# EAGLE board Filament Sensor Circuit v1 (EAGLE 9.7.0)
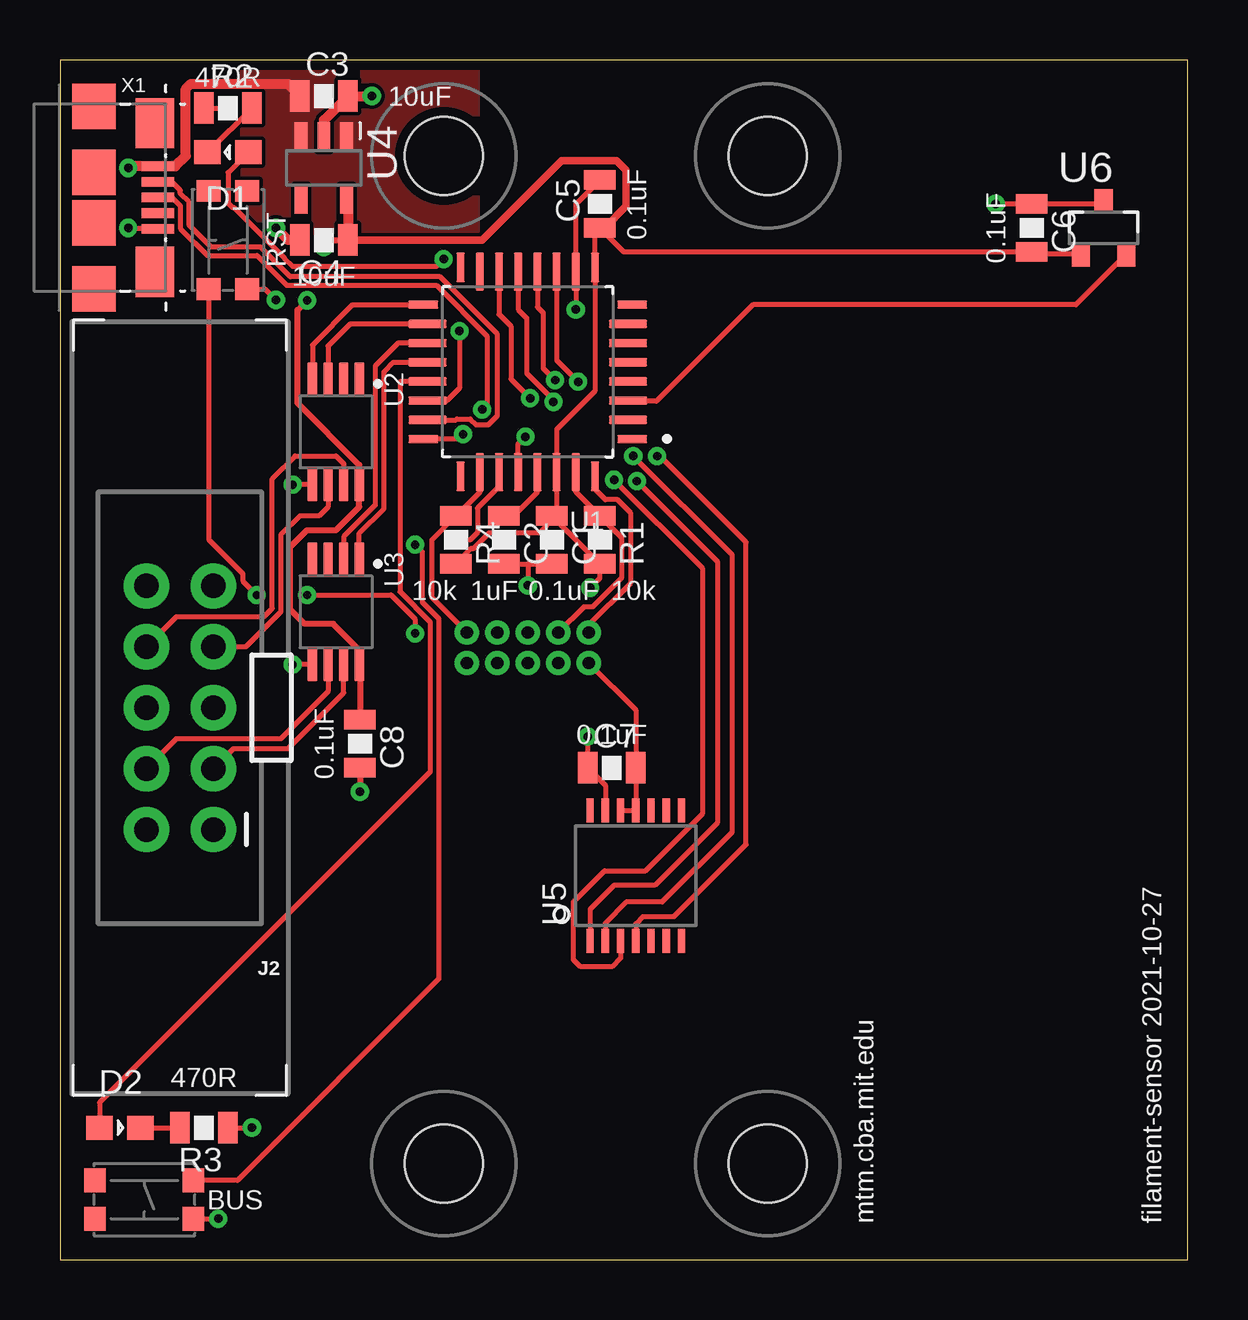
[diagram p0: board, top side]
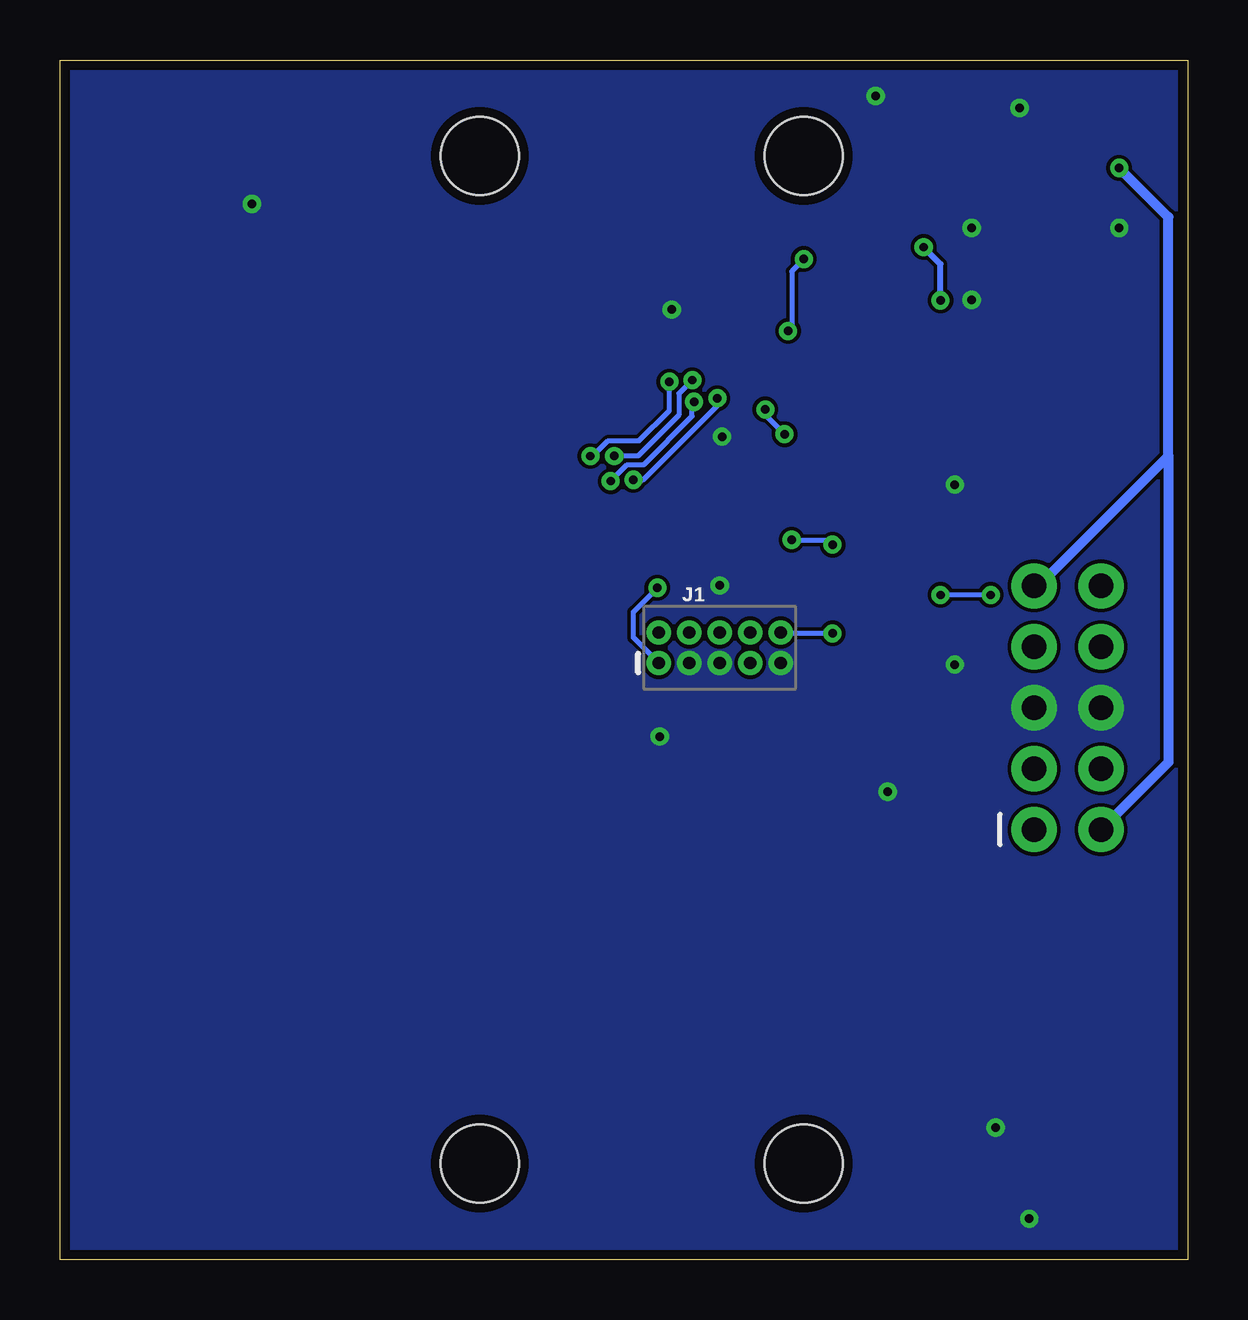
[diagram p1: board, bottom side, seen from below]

Size 47 x 50 mm. Coordinates in mm from the lower left corner, seen from the top.
Outline: 0,0 47,0 47,50 0,50 0,0
Copper layers (1*16): Top 0.035mm / dielectric 1.5mm / Bottom 0.035mm
Design rules "default *": minimum track width 6mil, minimum drill 0.35mm, track to track 6mil, track to pad 6mil, pad to pad 6mil, via to via 6mil, smd to smd 6mil, copper to edge 16mil, drill to drill 6mil, minimum pad ring 10mil, minimum via ring 8mil, stop-mask expansion 4mil, vias tented up to drill 40mil, thermal gap 10mil
Holes 3.25 mm at 16,46 29.5,46 16,4 29.5,4

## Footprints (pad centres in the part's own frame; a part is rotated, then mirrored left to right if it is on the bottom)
0805 = smd 0.8 x 1.3: 1 -1,0; 2 1,0
LED0805 = smd 1.1 x 1: 1 -0.85,0; 2 0.85,0
2X5-PTH-1.27MM = drill 0.508 pad 1: 1 -2.54,-0.635; 2 -2.54,0.635; 3 -1.27,-0.635; 4 -1.27,0.635; 5 0,-0.635; 6 0,0.635; 7 1.27,-0.635; 8 1.27,0.635; 9 2.54,-0.635; 10 2.54,0.635
2X5-SHROUDED_LOCK_LATCH = drill 1.016 pad 1.88: 1 -1.397,5.08; 2 1.397,5.08; 3 -1.397,2.54; 4 1.397,2.54; 5 -1.397,0; 6 1.397,0; 7 -1.397,-2.54; 8 1.397,-2.54; 9 -1.397,-5.08; 10 1.397,-5.08
TACT-SWITCH-KMR6 = smd 0.9 x 1: P$1 -2.05,0.8; P$2 2.05,0.8; P$3 -2.05,-0.8; P$4 2.05,-0.8
TQFP-32-FAB = smd 1.25 x 0.35: 1 -4.355,2.8; 8 -4.355,-2.8; 17 4.355,-2.8; 24 4.355,2.8 | smd 1.6 x 0.35: 2 -4.18,2; 3 -4.18,1.2; 4 -4.18,0.4; 5 -4.18,-0.4; 6 -4.18,-1.2; 7 -4.18,-2; 18 4.18,-2; 19 4.18,-1.2; 20 4.18,-0.4; 21 4.18,0.4; 22 4.18,1.2; 23 4.18,2 | smd 0.35 x 1.25: 9 -2.8,-4.355; 16 2.8,-4.355; 25 2.8,4.355; 32 -2.8,4.355 | smd 0.35 x 1.6: 10 -2,-4.18; 11 -1.2,-4.18; 12 -0.4,-4.18; 13 0.4,-4.18; 14 1.2,-4.18; 15 2,-4.18; 26 2,4.18; 27 1.2,4.18; 28 0.4,4.18; 29 -0.4,4.18; 30 -1.2,4.18; 31 -2,4.18
8-MSOP = smd 1.4 x 0.4: 1 -2.2,0.975; 2 -2.2,0.325; 3 -2.2,-0.325; 4 -2.2,-0.975; 5 2.2,-0.975; 6 2.2,-0.325; 7 2.2,0.325; 8 2.2,0.975
SOT23-5 = smd 0.533 x 1.194: 1 -0.95,-1.306; 2 0,-1.306; 3 0.95,-1.306; 4 0.95,1.306; 5 -0.95,1.306
TSSOP14 = smd 0.305 x 0.991: 1 -1.905,-2.718; 2 -1.27,-2.718; 3 -0.635,-2.718; 4 0,-2.718; 5 0.635,-2.718; 6 1.27,-2.718; 7 1.905,-2.718; 8 1.905,2.718; 9 1.27,2.718; 10 0.635,2.718; 11 0,2.718; 12 -0.635,2.718; 13 -1.27,2.718; 14 -1.905,2.718
SOT23 = smd 0.762 x 1.016: 1 -0.95,-1.1; 2 0.95,-1.1; 3 0,1.1
USB_MICRO_609-4613-1-ND = smd 0.4 x 1.35: D+ 0,2.675; D- -0.65,2.675; GND 1.3,2.675; ID 0.65,2.675; VBUS -1.3,2.675 | smd 1.9 x 1.8: HD0 -3.8,0; HD1 -1.05,0; HD2 1.05,0; HD3 3.8,0 | smd 2.1 x 1.6: HD4 -3.1,2.55; HD5 3.1,2.55

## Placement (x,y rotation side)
C1  0.1uF  [0805]  20.5,30 270 top
C2  1uF  [0805]  18.5,30 270 top
C3  10uF  [0805]  11,48.5 0 top
C4  10uF  [0805]  11,42.5 180 top
C5  0.1uF  [0805]  22.5,44 90 top
C6  0.1uF  [0805]  40.5,43 270 top
C7  0.1uF  [0805]  23,20.5 0 top
C8  0.1uF  [0805]  12.5,21.5 270 top
D1  LED0805  [LED0805]  7,46.15 180 top
D2  LED0805  [LED0805]  2.5,5.5 0 top
J1  CORTEX_DEBUG_PTH  [2X5-PTH-1.27MM]  19.5,25.5 0 bottom
J2  [2X5-SHROUDED_LOCK_LATCH]  5,23 180 top
R1  10k  [0805]  22.5,30 270 top
R2  470R  [0805]  7,48 0 top
R3  470R  [0805]  6,5.5 180 top
R4  10k  [0805]  16.5,30 270 top
S1  2-8X4-5_SWITCH  [TACT-SWITCH-KMR6]  7,42.5 270 top
S2  2-8X4-5_SWITCH  [TACT-SWITCH-KMR6]  3.52,2.5 0 top
U1  ATSAMD21E18A-AFFAB  [TQFP-32-FAB]  19.5,37 180 top
U2  RS485-ISL83078EMSOP  [8-MSOP]  11.5,34.5 270 top
U3  RS485-ISL83078EMSOP  [8-MSOP]  11.5,27 270 top
U4  VREG-AP2112  [SOT23-5]  11,45.5 180 top
U5  AS5047  [TSSOP14]  24,16 0 top
U6  HALLSOT23  [SOT23]  43.5,43 0 top
X1  USB  [USB_MICRO_609-4613-1-ND]  1.42,44.27 270 top

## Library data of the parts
C1-C8 R1-R4 = passives; PACKAGE: 0805
D1 D2 = lights
J1 J2 = SparkFun-Connectors
S1 S2 = passives
U1 = microcontrollers
U2 U3 = comm
U4 = power
U5 U6 = sensor
X1 = connector

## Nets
0-0-MOSI: U1.11 U5.4
0-1-CLK: U1.12 U5.2
0-2-CS: U1.13 U5.1
0-3-MISO: U1.14 U5.3
+3V3: C1.1 C4.1 C5.1 C6.2 C7.2 C8.1 J1.1 R1.2 R4.2 U1.9 U1.30 U2.8 U3.8 U4.5 U5.11 U5.12 U6.1
+5V: C3.1 J2.2 J2.9 U4.1 U4.3 X1.VBUS
A: J2.4 U3.6
B: J2.3 U3.7
GND: C1.2 C2.2 C3.2 C4.2 C5.2 C6.1 C7.1 C8.2 J1.3 J1.5 J1.9 J2.5 J2.6 R2.1 R3.1 S1.P$2 S2.P$4 U1.10 U1.28 U2.5 U3.5 U4.2 U5.13 U6.3 X1.GND
HALL: U1.3 U6.2
LIGHT: D1.1 U1.22
N$1: D1.2 R2.2
N$2: D2.2 R3.2
N$5: C2.1 U1.29
RESET: J1.10 R4.1 S1.P$4 U1.26
SWDCLK: J1.4 R1.1 U1.31
SWDIO: J1.2 U1.32
UCBUS_B: S2.P$2 U1.27
UCBUS_DE: U1.18 U2.3
UCBUS_L: D2.1 U1.21
UCBUS_RE: U1.19 U3.2
UCBUS_RX: U1.20 U3.1
UCBUS_TX: U1.17 U2.4
USBDM: U1.23 X1.D-
USBDP: U1.24 X1.D+
Y: J2.7 U2.6
Z: J2.8 U2.7

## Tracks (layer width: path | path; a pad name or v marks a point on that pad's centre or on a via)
0-0-MOSI  (via drill 0.35)
  Top 0.203: U1.11 20.7,37.49 v21.6,36.59 | v24.89,33.49 25.01,33.49 28.6,29.9 28.6,17.3 25.6,14.3 24.3,14.3 24,14 U5.4
  Bottom 0.203: v24.89,33.49 24.79,33.49 24.16,34.13 22.86,34.13 21.6,35.38 v21.6,36.59
0-1-CLK  (via drill 0.35)
  Top 0.203: U1.12 19.9,39.71 20.14,39.46 20.14,37.15 v20.64,36.66 | v23.89,33.49 28,29.39 28,17.8 25.1,14.9 23.6,14.9 22.73,14.03 U5.2
  Bottom 0.203: v20.64,36.66 21.2,36.1 21.2,35.2 22.91,33.49 v23.89,33.49
0-2-CS  (via drill 0.35)
  Top 0.203: U1.13 19.1,39.6 19.46,39.25 19.46,36.94 20.57,35.83 v20.57,35.75 | v24.05,32.45 27.4,29.09 27.4,18.2 24.8,15.6 23.1,15.6 22.09,14.6 U5.1
  Bottom 0.203: v24.05,32.45 | v24.05,32.45 23.36,33.13 22.66,33.13 20.65,35.15 20.65,35.67 v20.57,35.75
0-3-MISO  (via drill 0.35)
  Top 0.203: U1.14 18.3,39.4 18.8,38.9 18.8,36.7 v19.6,35.9 | U5.3 23.37,12.56 23,12.2 21.7,12.2 21.4,12.5 21.4,14.9 22.7,16.2 24.4,16.2 26.8,18.6 26.8,28.8 v23.1,32.5
  Bottom 0.203: v23.1,32.5 22.7,32.5 19.6,35.6 v19.6,35.9
+3V3  (via drill 0.35)
  Top 0.203: C5.1 22.3,42.8 U1.9 22.3,36.2 20.7,34.6 U1.30 20.7,31.2 C1.1 20.6,30.9 | 20.6,30.9 R1.2 22.5,28.4 v22.1,28 | 20.6,30.9 20,30.3 17.9,30.3 17.25,29.64 17.14,29.64 R4.2 | J1.1 24,22.91 C7.2 U5.11 U5.12 | 22.7,43 C5.1 | C5.1 23.5,42 C6.2 40.6,41.9 U6.1
  Top 0.254: v10.3,39.98 9.9,39.58 9.9,35.7 12.47,33.12 U2.8 12.47,31.38 11.5,30.4 10.3,30.4 9.6,29.7 9.6,27.1 10.2,26.5 11.39,26.5 12.47,25.42 U3.8 12.5,24.77 C8.1 | v11,42.2 11.3,42.5 C4.1
  Top 0.305: C4.1 17.6,42.5 20.9,45.8 23.2,45.8 23.6,45.4 23.6,43.9 22.7,43
  Top 0.406: U4.5 12,44.14 C4.1
  Bottom 0.203: J1.1 23.1,25.93 23.1,27 v22.1,28
  Bottom 0.254: v10.3,39.98 10.3,41.5 v11,42.2
+5V  (via drill 0.35)
  Top 0.406: C3.1 9.49,49.01 5.45,49.01 5.24,48.8 5.24,46 4.81,45.57 X1.VBUS 2.91,45.57 v2.85,45.5
  Bottom 0.406: J2.9 6.22,28.08 0.8,33.5 | 0.8,33.5 0.8,20.72 J2.2 | 0.8,33.5 0.8,43.45 v2.85,45.5
  pour Top (no thermals): 7.7,42.7 17.3,42.7 17.3,50.3 7.7,50.3
A
  Top 0.203: U3.6 11.18,23.68 9.2,21.7 4.84,21.7 J2.4
B
  Top 0.203: J2.3 7.24,21.3 9.5,21.3 11.82,23.62 U3.7
GND  (via drill 0.35)
  Top 0.203: S1.P$2 8.55,40.45 v9,40 | R2.1 v7,48 | U2.5 v9.7,32.3 | U3.5 v9.7,24.8 | R3.1 v8,5.5 | S2.P$4 v6.6,1.7 | C5.2 21.5,44 U1.10 v21.5,39.6 | U1.28 19.1,34 v19.4,34.3 | C2.2 19.5,29 | 19.5,29 C1.2 | 19.5,29 v19.5,28.1 | v22,21.8 C7.1 22.73,19.77 U5.13 22.7,18.75 | X1.GND 2.88,42.97 v2.85,43 | U6.3 43.4,44 C6.1 v39,44
  Top 0.254: C8.2 v12.5,19.5
  Top 0.406: U4.2 11,47.5 C3.2 v13,48.5 | C4.2 9.5,42.5 v9,43
  pour Bottom (no thermals): -0.9,-0.9 48.4,-0.9 48.4,50.9 -0.9,50.9
HALL
  Top 0.203: U6.2 42.35,39.8 28.89,39.8 24.86,35.77 23.71,35.77 U1.3
LIGHT  (via drill 0.35)
  Top 0.203: D1.1 7,45.3 7,44.04 7.2,43.85 7.25,43.85 9.35,41.75 9.35,41.74 9.69,41.4 15.69,41.4 v15.99,41.7 | v16.65,38.7 16.65,36.32 16.13,35.8 U1.22
  Bottom 0.203: v15.99,41.7 16.5,41.19 16.5,38.85 v16.65,38.7
N$1
  Top 0.203: R2.2 D1.2
N$2
  Top 0.203: D2.2 R3.2
N$5
  Top 0.203: U1.29 19.9,32 18.9,31 C2.1
RESET  (via drill 0.35)
  Top 0.203: J1.10 15.5,27.59 15.5,30 16.45,30.95 R4.1 17.5,32 U1.26 | v8.2,27.7 7.62,28.28 7.62,28.59 6.2,30 S1.P$4 | v10.3,27.7 13.8,27.7 14.8,26.7 v14.8,26.1
  Bottom 0.203: v8.2,27.7 v10.3,27.7 | v14.8,26.1 16.93,26.1 J1.10
SWDCLK
  Top 0.203: U1.31 21.5,32 R1.1 23.4,30.1 23.4,28.4 22.2,27.2 21.84,27.2 J1.4
SWDIO
  Top 0.203: J1.2 22.04,26.44 23.8,28.2 23.8,31.11 23.24,31.67 22.74,31.67 22.3,32.11 U1.32
UCBUS_B  (via drill 0.35)
  Top 0.203: S2.P$2 7.4,3.3 15.79,11.69 15.79,26.72 15.1,27.41 15.1,29.5 v14.8,29.8 | U1.27 18.3,32.21 17.4,31.31 17.4,30.3 17.1,30 v16.5,30
  Bottom 0.203: v16.5,30 15,30 v14.8,29.8
UCBUS_DE
  Top 0.203: U1.18 12.1,39 11.18,38.08 U2.3
UCBUS_L
  Top 0.203: U1.21 14.2,36.6 14.17,36.57 14.17,27.84 15.43,26.57 15.43,20.33 1.65,6.55 D2.1
UCBUS_RE
  Top 0.203: U1.19 14.1,38.2 13.14,37.24 13.14,31.45 11.82,30.13 U3.2
UCBUS_RX
  Top 0.203: U3.1 12.47,30.27 13.5,31.3 13.5,37 13.9,37.4 U1.20
UCBUS_TX
  Top 0.203: U1.17 12.2,39.8 10.53,38.12 U2.4
USBDM
  Top 0.203: X1.D- 4.67,44.92 5.02,44.57 5.02,44.42 5.38,44.07 5.38,43.12 6.3,42.2 8.36,42.2 9.6,40.97 15.84,40.97 18.23,38.57 18.23,35.17 17.86,34.8 17.34,34.8 17.1,35.03 16.54,35.03 16.51,35 U1.23
USBDP  (via drill 0.35)
  Top 0.203: X1.D+ 4.67,44.27 5.02,43.92 5.02,42.98 6.15,41.84 8.21,41.84 9.45,40.61 15.69,40.61 17.8,38.5 17.8,35.63 v17.6,35.43 | v16.8,34.4 16.6,34.2 U1.24
  Bottom 0.203: v17.6,35.43 17.6,35.2 v16.8,34.4
Y
  Top 0.203: U2.6 11.18,31.38 10.8,31 10,31 9.2,30.2 9.2,27 7.74,25.54 J2.7
Z
  Top 0.203: J2.8 4.86,26.8 8.5,26.8 8.84,27.14 8.84,32.54 9.8,33.5 11.5,33.5 11.82,33.17 U2.7

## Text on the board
tPlace: RST | BUS | mtm.cba.mit.edu | filament-sensor 2021-10-27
